PROGRAM MAIN
VAR CONSTANT
    cInitSource				: ST_MA_MultiArray_InitPars := ( eTypeCode := eMA_TypeCode_LREAL, nDims := 2, aDimSizes := [cChannels, cBufferLength]);
END_VAR

VAR
	(* Input *)	
	nInputSelection			: UDINT := 1;						// Switch between hardware and function generator	
	nSample					: UDINT;
	// Hardware
	aEl3632Ch1 AT %I*		: ARRAY[1..cOversamples] OF INT;	// Input from hardware e.g. EL3632 ch1
	aEl3632Ch2 AT %I*		: ARRAY[1..cOversamples] OF INT;	// Input from hardware e.g. EL3632 ch2
	// Function generator
	fbFunctionGenerator1	: FB_FunctionGenerator;				// Signal Generator, ch1
	fSetFrequency1			: LREAL := 400;		        		// Hz
	fSetAmplitude1			: LREAL := 4;		        		// peak amplitude of sin signal [m/s^2]
	fbFunctionGenerator2	: FB_FunctionGenerator;				// Signal Generator, ch2
	fSetFrequency2			: LREAL := 35;		        		// Hz
	fSetAmplitude2			: LREAL := 4;		        		// peak amplitude of sin signal	[m/s^2]	
	
	(* Input from aBuffer to fbSource *)
	aBuffer					: ARRAY[1..cChannels] OF ARRAY[1..cOversamples] OF LREAL;						
	fbSource				: FB_CMA_Source :=(	stInitPars := cInitSource, nOwnID := eID_Source, aDestIDs := [eID_VA]);		// Initialize source buffers
								
	(* From fbSink to aVAResult *)	
	fbSink					: FB_CMA_Sink := (nOwnID := eID_Sink);
	// Results for each configured band: [ class, order, channel ]
	aVAResult   			: ARRAY[1..cMaxBands] OF ARRAY[1..3] OF DINT;
	
	(* Handle Results *)
	nCountResults			: ULINT;	
	bCalculate				: BOOL;
	
	(* Error monitoring *)
	fbErrHist				: FB_HRErrHist; 

	(* output *)
	ISO_10816_nSelectedBand			: UDINT := 1;			// Select Frequency range for classification
	ISO_10816_HighscoreClass AT%Q* 	: E_IsoClass;
	ISO_10816_HighscoreOrder		: DINT;	
	ISO_10816_HighscoreChannel		: DINT;
	
END_VAR

(* Input *)
CASE nInputSelection OF
	0:  (* input from EL3632 *)
		FOR nSample := 1 TO cOversamples DO
			aBuffer[1][nSample] := cScale*INT_TO_LREAL(aEl3632Ch1[nSample]); // convert from Volts to acceleration in m/s^2
			aBuffer[2][nSample] := cScale*INT_TO_LREAL(aEl3632Ch2[nSample]);
		END_FOR 
	1:  (* signal generator *)		
		fbFunctionGenerator1(	fFrequency 	:= fSetFrequency1,
								fAmplitude 	:= fSetAmplitude1,
								eFunction 	:= E_FunctionType.Sine,
								aSignal		:= aBuffer[1] );	
		fbFunctionGenerator2(	fFrequency 	:= fSetFrequency2,
								fAmplitude 	:= fSetAmplitude2,
								eFunction 	:= E_FunctionType.Sine,
								aSignal		:= aBuffer[2] );	
END_CASE					

(* Call source to collect data *)
fbSource.Input2DStd(pDataIn 		:= ADR(aBuffer),
					nDataInSize 	:= SIZEOF(aBuffer), 
					eElementType 	:= eMA_TypeCode_LREAL,
					nOptionPars		:= cCMA_Option_MarkInterruption ); 
IF fbSource.bError THEN
	fbErrHist.AddError(bErr:=TRUE, hrErrCode:=fbSource.hrErrorCode, sErrSource:='MAIN.fbSource'); // error monitoring
	// ToDo: if error
END_IF

(* Push results to sink *)
fbSink.Output1DStd(	pDataOut 		:= ADR(aVAResult), 
					nDataOutSize 	:= SIZEOF(aVAResult), 
					eElementType 	:= eMA_TypeCode_INT32, 
					nOptionPars		:= 0,
					bNewResult		=> bCalculate );
IF fbSink.bError THEN
	fbErrHist.AddError(bErr:=TRUE, hrErrCode:=fbSink.hrErrorCode, sErrSource:='MAIN.fbSink'); // error monitoring
	// ToDo: if error
END_IF

// define class according to ISO 10816-3 based on velocity and displacement data for each measurement channel
IF bCalculate THEN	
	// Highscore in classification according to ISO 10816-3.
	ISO_10816_HighscoreClass 	:= aVAResult[ISO_10816_nSelectedBand][1];		// class
	ISO_10816_HighscoreOrder 	:= aVAResult[ISO_10816_nSelectedBand][2];		// order
	ISO_10816_HighscoreChannel	:= aVAResult[ISO_10816_nSelectedBand][3];		// channel

	IF NOT (ISO_10816_HighscoreClass = E_IsoClass.Error) THEN 
		nCountResults := fbSink.nCntResults;
		// ToDo: if succeeded
	ELSE
		// ToDo: if error; RMS result is NaN... code here what to do.
	END_IF;
END_IF

END_PROGRAM
